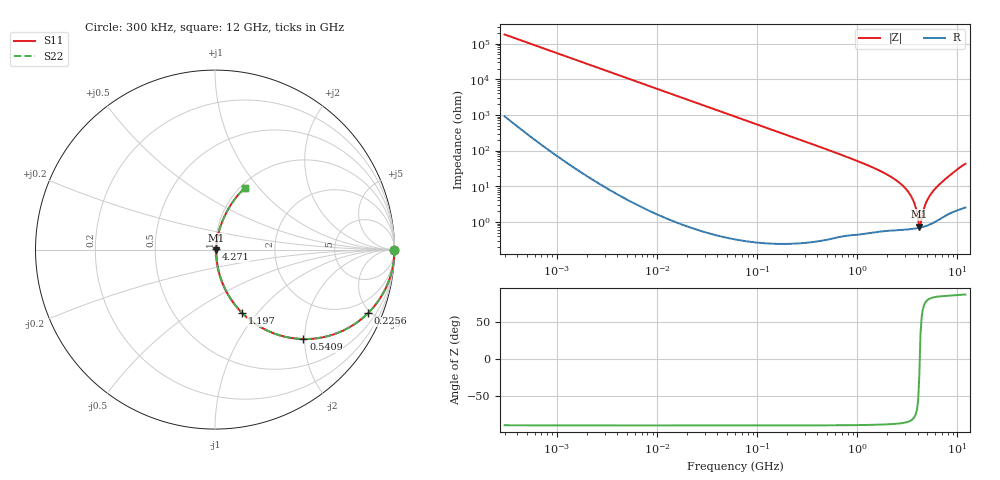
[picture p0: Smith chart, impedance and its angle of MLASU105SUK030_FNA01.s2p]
! MLASU105SUK030_FNA01  S-PARAMETER MODEL  ( General Type )
! Model Generated by TAIYO YUDEN Corporation (http://www.ty-top.com)
! Version 2.0
! TAIYO YUDEN Control No. 120810
! Copyright(c) 2011 TAIYO YUDEN CO.,LTD. All Rights Reserved.
! Product Description (link to TY-COMPAS)
! https://ds.yuden.co.jp/TYCOMPAS/or/detail?pn=MLASU105SUK030CFNA01&u=M
! Products Name : Multilayer Ceramic Capacitors
! Characteristics :
!  Capacitance : 3 pF , Rated Voltage : 50V , TCC : UK / U2K
!  Case Size : 1.0 x 0.5 / 0.039 x 0.02 [mm/inch] , Thickness : 0.5 / 0.02 [mm/inch]
!  (Conditions: Temperature = 25 degC , DC Bias Current/Voltage = 0A / 0V)
! External Node Assignments :
!  1  o---| |---o  2
! GND o---------o GND
! Frequency Range : 0.3MHz  -  12000MHz  [ 401 STEP ]
# MHz S RI R 50
! Freq[MHz].  S11 Real  S11 Imag  S21 Real  S21 Imag  S12 Real  S12 Imag  S22 Real  S22 Imag
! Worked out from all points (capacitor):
!   401 points, 300 kHz to 12 GHz, reference 50 ohm
!   read as one part in series: C = 2.94 pF near 316.3 kHz
!   lowest |Z| = 741 mohm at 4.159 GHz (marker M1)
!   series resonance near 4.203 GHz, so ESL is about 490 pH
!   S11 on the Smith chart (normalised r, x): 300 kHz: open; 225.6 MHz: 1.00, -4.79; 540.9 MHz: 1.01, -1.97; 1.197 GHz: 1.01, -0.83; 4.271 GHz: 1.01, +0.01; 12 GHz: 1.05, +0.85
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0.3  1 -0.000553  3.1e-06 0.000553  3.1e-06 0.000553  1 -0.000553
1.769972  1 -0.00327  1.32e-05 0.00327  1.32e-05 0.00327  1 -0.00327
10.44266  0.9996 -0.0193  0.000377 0.0193  0.000377 0.0193  0.9996 -0.0193
60  0.9878 -0.1094  0.0122 0.1094  0.0122 0.1094  0.9878 -0.1094
129.3602  0.9459 -0.2259  0.0541 0.2259  0.0541 0.2259  0.9459 -0.2259
225.6362  0.8513 -0.3553  0.1487 0.3553  0.1487 0.3553  0.8513 -0.3553
353.9943  0.6977 -0.4584  0.3023 0.4584  0.3023 0.4584  0.6977 -0.4584
540.8523  0.4928 -0.4983  0.5072 0.4983  0.5072 0.4983  0.4928 -0.4983
763.2128  0.3215 -0.4641  0.6785 0.4641  0.6785 0.4641  0.3215 -0.4641
1197.383  0.1504 -0.3518  0.8496 0.3518  0.8496 0.3518  0.1504 -0.3518
2088.533  0.0419 -0.1864  0.9581 0.1864  0.9581 0.1864  0.0419 -0.1864
2722.03  0.0189 -0.113  0.9811 0.113  0.9811 0.113  0.0189 -0.113
3276.641  0.0103 -0.0642  0.9897 0.0642  0.9897 0.0642  0.0103 -0.0642
3642.919  0.00776 -0.0369  0.9922 0.0369  0.9922 0.0369  0.00776 -0.0369
4050.141  0.00679 -0.00983  0.9932 0.00983  0.9932 0.00983  0.00679 -0.00983
4158.869  0.0068 -0.00282  0.9932 0.00282  0.9932 0.00282  0.0068 -0.00282
4270.516  0.00691 0.00438  0.9931 -0.00438  0.9931 -0.00438  0.00691 0.00438
4385.161  0.00712 0.0101  0.9929 -0.0101  0.9929 -0.0101  0.00712 0.0101
4875.354  0.00881 0.034  0.9912 -0.034  0.9912 -0.034  0.00881 0.034
5715.274  0.0144 0.0712  0.9856 -0.0712  0.9856 -0.0712  0.0144 0.0712
8064.993  0.0472 0.1724  0.9528 -0.1724  0.9528 -0.1724  0.0472 0.1724
12000  0.168 0.3452  0.832 -0.3452  0.832 -0.3452  0.168 0.3452
